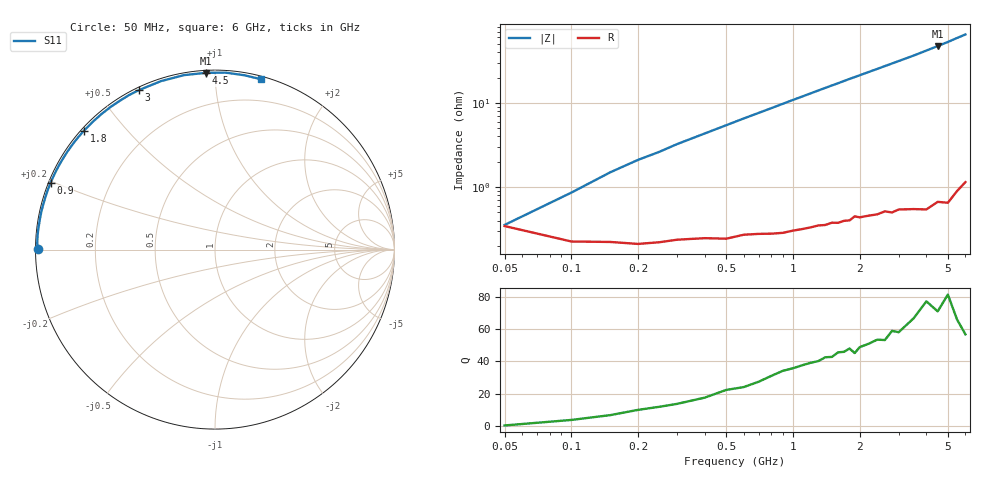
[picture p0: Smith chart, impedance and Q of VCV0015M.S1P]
! Infineon Technologies  Discrete & RF Semiconductors
! BBY 56-03
! Si Tuning Diode in SOD323
! VR =
! S-Parameters:  June  1999
# GHz  S  MA  R  50
!  f  S11
! GHz  MAG  ANG
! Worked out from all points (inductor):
!   34 points, 50 MHz to 6 GHz, reference 50 ohm
!   read as one part to ground: L = 1.57 nH near 100 MHz
!   highest Q = 77.3 at 4.5 GHz (marker M1), where L = 1.68 nH
!   S11 on the Smith chart (normalised r, x): 50 MHz: 0.01, +0.00; 900 MHz: 0.01, +0.20; 1.8 GHz: 0.01, +0.39; 3 GHz: 0.01, +0.63; 4.5 GHz: 0.01, +0.95; 6 GHz: 0.02, +1.30
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0.05  0.9863 179.8
0.1  0.991 178.1
0.2  0.9916 175.2
0.25  0.9912 174.0
0.3  0.9906 172.6
0.4  0.9902 170.1
0.5  0.9904 167.6
0.6  0.9894 165.1
0.8  0.9892 160.3
0.9  0.989 157.9
1  0.9885 155.5
1.1  0.9881 153.2
1.3  0.9871 148.6
1.5  0.9864 144.2
1.6  0.9866 142.1
1.8  0.9861 137.8
2  0.9853 133.8
2.2  0.9851 129.9
2.4  0.985 126.2
2.6  0.9843 122.5
2.8  0.9853 119.0
3  0.9846 115.6
3.5  0.9858 107.7
4  0.9873 100.0
4.5  0.986 93.0
5  0.9878 86.6
5.5  0.9852 80.4
6  0.9831 75.0
